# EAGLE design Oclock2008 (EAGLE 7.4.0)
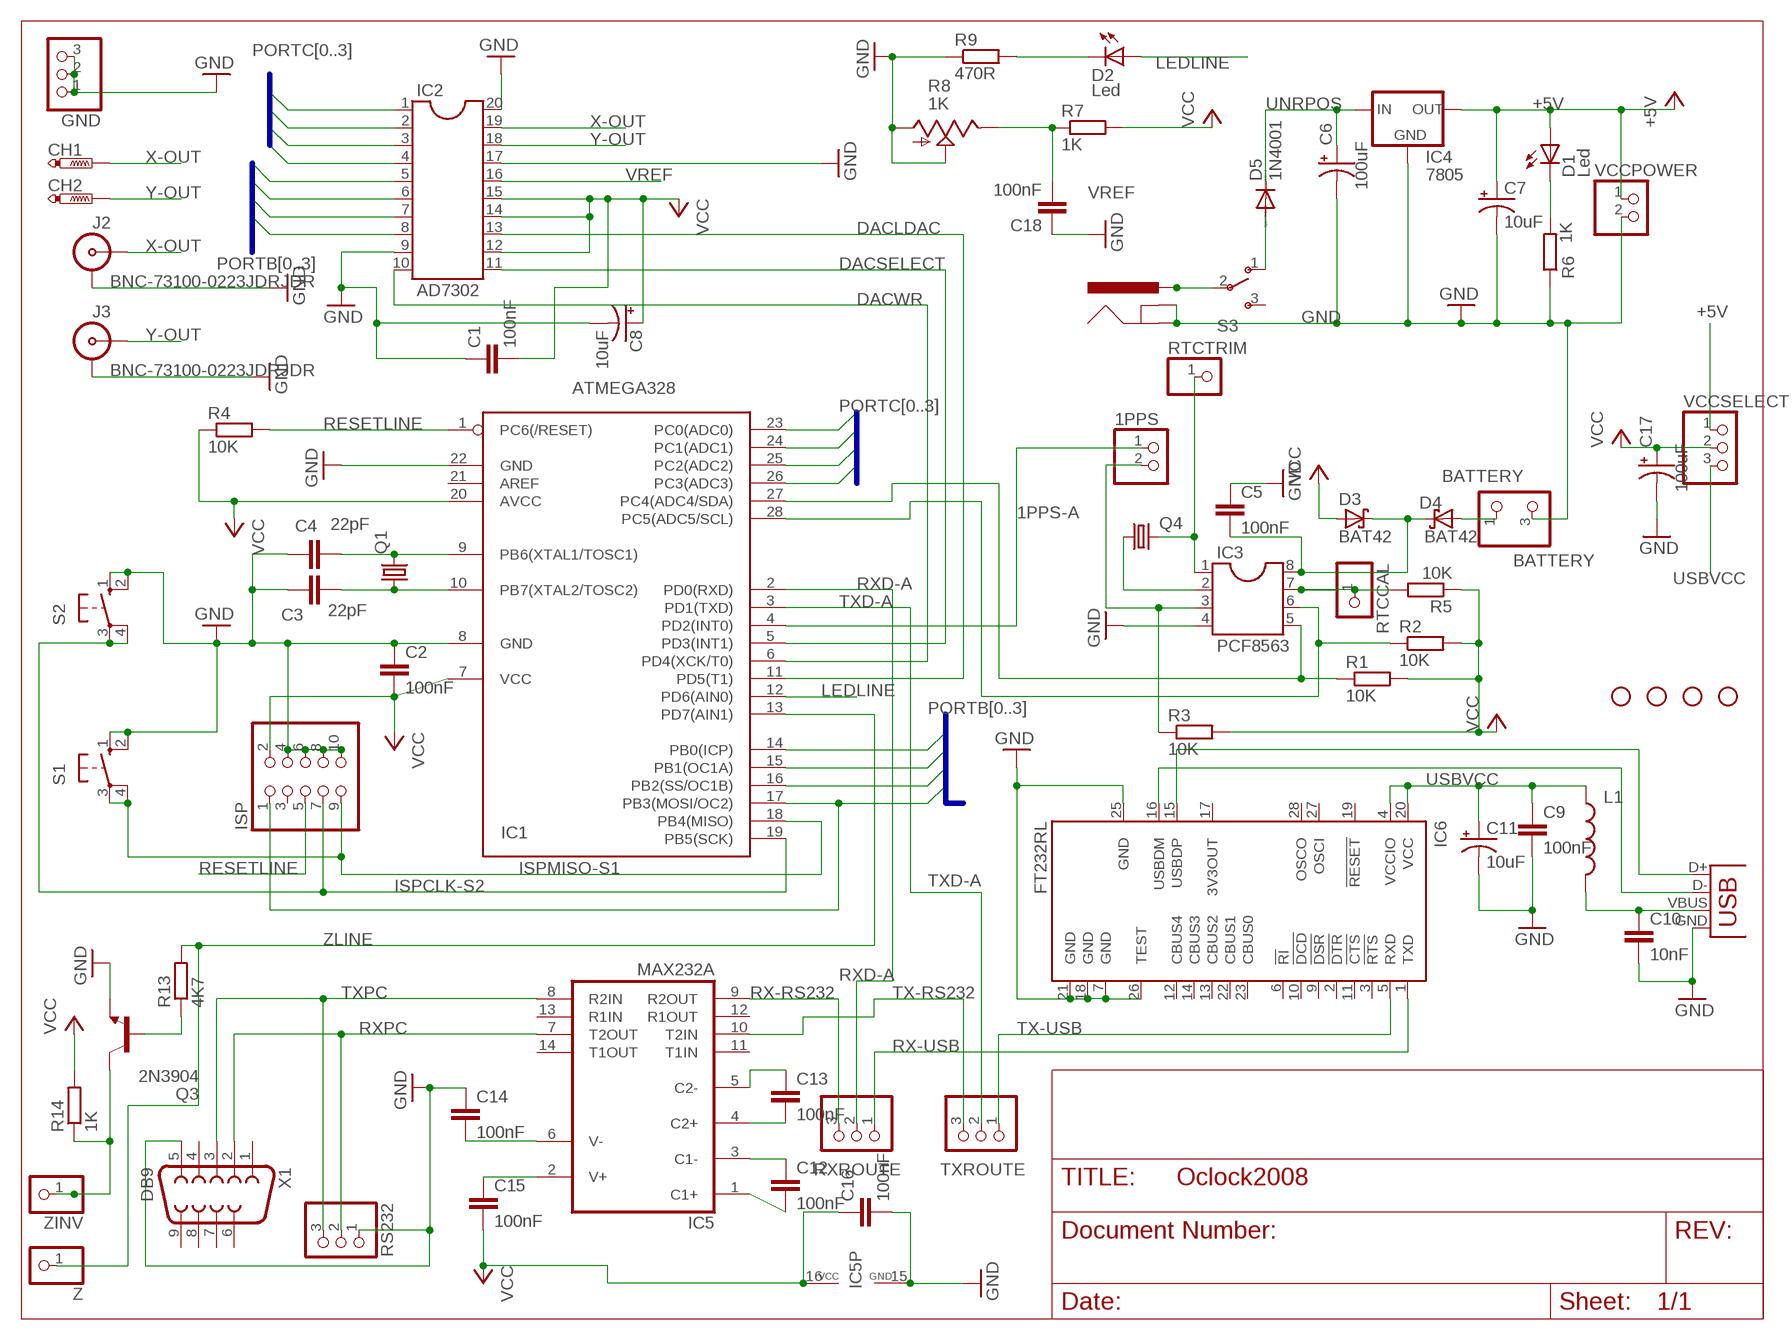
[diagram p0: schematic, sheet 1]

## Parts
1PPS  PINHD-1X2  [1X02]
BATTERY  BATTERY  PINHD-1X3BAT  [1X03BAT]
C1  100nF  C-EU025-025X050  [C025-025X050]
C2  100nF  C-EU025-025X050  [C025-025X050]
C3  22pF  C-EU025-025X050  [C025-025X050]
C4  22pF  C-EU025-025X050  [C025-025X050]
C5  100nF  C-EU025-025X050  [C025-025X050]
C6  100uF  CPOL-USE2.5-7  [E2,5-7]
C7  10uF  CPOL-USE2.5-5  [E2,5-5]
C8  10uF  CPOL-USE2.5-5  [E2,5-5]
C9  100nF  CAP0603  [0603]
C10  10nF  CAP0603  [0603]
C11  10uF  CAP_POL3528  [EIA3528]
C12  100nF  C-EU025-025X050  [C025-025X050]
C13  100nF  C-EU025-025X050  [C025-025X050]
C14  100nF  C-EU025-025X050  [C025-025X050]
C15  100nF  C-EU025-025X050  [C025-025X050]
C16  100nF  C-EU025-025X050  [C025-025X050]
C17  100uF  CPOL-USE2.5-7  [E2,5-7]
C18  100nF  C-EU025-025X050  [C025-025X050]
CH1  PTR1PAD1-20Y  [P1-20Y]
CH2  PTR1PAD1-20Y  [P1-20Y]
D1  Led  LED3MM  [LED3MM]
D2  Led  LED3MM  [LED3MM]
D3  BAT42  SCHOTTKY-DIODEDO35-7  [DO35-7]
D4  BAT42  SCHOTTKY-DIODEDO35-7  [DO35-7]
D5  1N4001  1N4004  [DO41-10]
GND  PINHD-1X3  [1X03]
IC1  ATMEGA328  MEGA8-P  [DIL28-3]
IC2  AD7302  DIL20  [DIL20]
IC3  PCF8563  DIL8  [DIL08]
IC4  7805  V_REG_78XXSINK  [TO220-IGO]
IC5  MAX232A  MAX232  [DIL16]
IC6  FT232RL  [SSOP28]
ISP  PINHD-2X5  [2X05]
J1  POWER_JACKPTH  [POWER_JACK_PTH]
J2  BNC-73100-0223JDRJDR  [73100-0223JDR]
J3  BNC-73100-0223JDRJDR  [73100-0223JDR]
L1  INDUCTOR0603  [0603]
Q1  CRYSTALHC18U-V  [HC18U-V]
Q3  2N3904  [TO92]
Q4  CRYSTALTC26H  [TC26H]
R1  10K  R-EU_0207/10  [0207/10]
R2  10K  R-EU_0207/10  [0207/10]
R3  10K  R-EU_0207/10  [0207/10]
R4  10K  R-EU_0207/10  [0207/10]
R5  10K  R-EU_0207/10  [0207/10]
R6  1K  R-EU_0207/10  [0207/10]
R7  1K  R-EU_0207/10  [0207/10]
R8  1K  TRIM_US-LI10  [LI10]
R9  470R  R-EU_0207/10  [0207/10]
R13  4K7  R-EU_0207/10  [0207/10]
R14  1K  R-EU_0207/10  [0207/10]
RS232  PINHD-1X3  [1X03]
RTCCAL  PINHD-1X1  [1X01]
RTCTRIM  PINHD-1X1  [1X01]
RXROUTE  PINHD-1X3  [1X03]
S1  10-XX  [B3F-10XX]
S2  10-XX  [B3F-10XX]
S3  SWITCH-SPSTPTH  [SWITCH-SPST]
TXROUTE  PINHD-1X3  [1X03]
U$2  STAND-OFF  [STAND-OFF]
U$3  STAND-OFF  [STAND-OFF]
U$4  STAND-OFF  [STAND-OFF]
U$5  STAND-OFF  [STAND-OFF]
VCCPOWER  PINHD-1X2  [1X02]
VCCSELECT  PINHD-1X3  [1X03]
X1  DB9  [DB9]
X2  USBPTH  [USB-B-PTH]
Z  PINHD-1X1  [1X01]
ZINV  PINHD-1X1  [1X01]

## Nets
1PPS-A: 1PPS.1 IC1.4(PD2(INT0))
1PPS-B: 1PPS.2 IC3.3 R3.1
+5V: C7.+ D1.A IC4.OUT VCCPOWER.1 VCCSELECT.1
BATPOWER: BATTERY.1 D4.A
DACLDAC: IC1.11(PD5(T1)) IC2.13
DACSELECT: IC1.5(PD3(INT1)) IC2.11
DACWR: IC1.6(PD4(XCK/T0)) IC2.10
GND: BATTERY.3 C1.1 C2.1 C3.2 C4.2 C5.1 C6.- C7.- C8.- C9.2 C10.2 C11.C(-) C14.1 C16.2 C17.- C18.1 GND.1 GND.2 GND.3 IC1.8(GND) IC1.22(GND) IC2.9 IC2.17 IC2.20 IC3.4 IC4.GND IC5.15(GND) IC6.7(GND) IC6.18(GND) IC6.21(GND) IC6.25(GND) IC6.26(TEST) ISP.4 ISP.6 ISP.8 ISP.10 J1.GND J1.GNDBREAK J2.GND J3.GND Q3.3(E) R6.1 R8.A R8.S R9.1 RS232.1 S1.1(S) S1.2(S1) S2.1(S) S2.2(S1) VCCPOWER.2 X1.5 X2.GND
ISPCLK-S2: IC1.19(PB5(SCK)) ISP.7 S2.3(P) S2.4(P1)
ISPMISO-S1: IC1.18(PB4(MISO)) ISP.9 S1.3(P) S1.4(P1)
LEDLINE: D2.A IC1.12(PD6(AIN0))
N$1: IC3.7 R5.2 RTCCAL.1
N$2: J1.PWR S3.2(P)
N$3: D2.K(C) R9.2
N$6: D1.K(C) R6.2
N$7: D5.A S3.1(O)
N$8: C13.2 IC5.4(C2+)
N$11: C4.1 IC1.9(PB6(XTAL1/TOSC1)) Q1.2
N$12: C3.1 IC1.10(PB7(XTAL2/TOSC2)) Q1.1
N$13: IC3.1 Q4.2 RTCTRIM.1
N$14: IC3.2 Q4.1
N$15: C13.1 IC5.5(C2-)
N$20: C12.1 IC5.3(C1-)
N$21: C12.2 IC5.1(C1+)
N$22: C14.2 IC5.6(V-)
N$23: C15.1 IC5.2(V+)
N$26: Q3.2(B) R13.1
PORTB0: IC1.14(PB0(ICP)) IC2.8
PORTB1: IC1.15(PB1(OC1A)) IC2.7
PORTB2: IC1.16(PB2(SS/OC1B)) IC2.6
PORTB3: IC1.17(PB3(MOSI/OC2)) IC2.5 ISP.1
PORTC0: IC1.23(PC0(ADC0)) IC2.4
PORTC1: IC1.24(PC1(ADC1)) IC2.3
PORTC2: IC1.25(PC2(ADC2)) IC2.2
PORTC3: IC1.26(PC3(ADC3)) IC2.1
RESETLINE: IC1.1(PC6(/RESET)) ISP.5 R4.2
RTCPOWER: C5.2 D3.C D4.C IC3.8
RX-RS232: IC5.9(R2OUT) RXROUTE.3
RX-USB: IC6.1(TXD) RXROUTE.1
RXD-A: IC1.2(PD0(RXD)) RXROUTE.2
RXPC: IC5.7(T2OUT) RS232.2 X1.2
SCLLINE: IC1.28(PC5(ADC5/SCL)) IC3.6 R2.1
SDALINE: IC1.27(PC4(ADC4/SDA)) IC3.5 R1.1
TX-RS232: IC5.10(T2IN) TXROUTE.3
TX-USB: IC6.5(RXD) TXROUTE.1
TXD-A: IC1.3(PD1(TXD)) TXROUTE.2
TXPC: IC5.8(R2IN) RS232.3 X1.3
UNRPOS: C6.+ D5.C IC4.IN
USB5V: C10.1 L1.2 X2.VBUS
USBDM: IC6.16(USBDM) X2.D-
USBDP: IC6.15(USBDP) X2.D+
USBVCC: C9.1 C11.A(+) IC6.4(VCCIO) IC6.20(VCC) L1.1 VCCSELECT.3
VCC: C1.2 C2.2 C8.+ C15.2 C16.1 C17.+ D3.A IC1.7(VCC) IC1.20(AVCC) IC2.12 IC2.14 IC2.15 IC5.16(VCC) ISP.2 R1.2 R2.2 R3.2 R4.1 R5.1 R7.2 R14.2 VCCSELECT.2
VREF: C18.2 IC2.16 R7.1 R8.E
X-OUT: CH1.TP IC2.19 J2.P
Y-OUT: CH2.TP IC2.18 J3.P
ZINVLINE: Q3.1(C) R14.1 ZINV.1
ZLINE: IC1.13(PD7(AIN1)) R13.2 Z.1
Unconnected: IC1.21(AREF) IC5.11(T1IN) IC5.12(R1OUT) IC5.13(R1IN) IC5.14(T1OUT) IC6.2(!DTR) IC6.3(!RTS) IC6.6(!RI) IC6.9(!DSR) IC6.10(!DCD) IC6.11(!CTS) IC6.12(CBUS4) IC6.13(CBUS2) IC6.14(CBUS3) IC6.17(3V3OUT) IC6.19(!RESET) IC6.22(CBUS1) IC6.23(CBUS0) IC6.27(OSCI) IC6.28(OSCO) ISP.3 S3.3(S) X1.1 X1.4 X1.6 X1.7 X1.8 X1.9

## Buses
PORTC[0..3]
PORTB[0..3]

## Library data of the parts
1PPS VCCPOWER = pinhead:PINHD-1X2: PIN HEADER
BATTERY = pinhead:PINHD-1X3BAT
C1-C5 C12-C16 C18 = rcl:C-EU: CAPACITOR, European symbol
C6-C8 C17 = rcl:CPOL-US: POLARIZED CAPACITOR, American symbol
C9 C10 = SparkFun:CAP: Capacitor
C11 = SparkFun:CAP_POL: Capacitor Polarized
CH1 CH2 = testpad:PTR1: TEST PIN
D1 D2 = led:LED: LED
D3 D4 = diode:SCHOTTKY-DIODE: Schottky Diode
D5 = diode:1N4004: DIODE
GND RS232 RXROUTE TXROUTE VCCSELECT = pinhead:PINHD-1X3: PIN HEADER
IC1 = atmel:MEGA8-P: MICROCONTROLLER 8 Kbytes FLASH, 1 kbytes SRAM, 512 bytes EEPROM, USART, 4-channel 10 bit ADC, 2-channel 8 bit ADC Pin compatible with Atmega48, ATMega88, ATMega168 Source: avr.lbr; OC_FARNELL: unknown; OC_NEWARK: unknown
IC2 = ic-package:DIL20: Dual In Line / Socket
IC3 = ic-package:DIL8: Dual In Line / Socket
IC4 = SparkFun:V_REG_78XX: Voltage Regulator Standard 7805 5V regulator. IGO (Input Ground Output). Spark Fun Electronics SKU : COM-00107
IC5 = maxim:MAX232: RS232 TRANSCEIVER; MF: MAXIM; MPN: MAX232ACPE+; OC_FARNELL: 9723773; OC_NEWARK: 68K4544
IC6 = ftdichip:FT232R: Source: http://www.ftdichip.com/Documents/DataSheets/DS_FT232R_v104.pdf; MPN: FT232RL; OC_FARNELL: 1146032; OC_NEWARK: 91K9918
ISP = pinhead:PINHD-2X5: PIN HEADER
J1 = SparkFun:POWER_JACK: Power Jack This is the standard 5.5mm barrel jack for power. The PTH is the most common, proven, reliable, footprint. All others are experimental. The Slot footprint only works if the mill layer is transmitted to the PCB fab house so be warned. Spark Fun Electronics SKU : PRT-00119. Mating wall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
J2 J3 = Jdr-Eagle:BNC-73100-0223JDR
L1 = SparkFun:INDUCTOR: Inductors
Q1 Q4 = crystal:CRYSTAL: CRYSTAL; OC_FARNELL: unknown; OC_NEWARK: unknown
Q3 = transistor-npn:2N3904: NPN Transistor
R1-R7 R9 R13 R14 = rcl:R-EU_: RESISTOR, European symbol
R8 = pot:TRIM_US-: POTENTIOMETER
RTCCAL RTCTRIM Z ZINV = pinhead:PINHD-1X1: PIN HEADER
S1 S2 = switch-omron:10-XX: OMRON SWITCH; MPN: B3F-1000; OC_FARNELL: 176432; OC_NEWARK: 36M3542
S3 = SparkFun:SWITCH-SPST: SPST Switch Simple slide switch. Spark Fun Electronics SKU : COM-00102
U$2-U$5 = SparkFun:STAND-OFF: Stand Off
X1 = SparkFun:DB9: DB9 Connector Standard DB9 (D-Sub 9) serial connector. Can be used for CAN bus as well as RS485 and RS232. Footprint production proven. Spark Fun Electronics SKU : PRT-00429
X2 = SparkFun:USB: USB Connectors USB-B-PTH is fully proven SKU : PRT-00139 USB-miniB is fully proven SKU : PRT-00587 USB-A-PCB is untested. USB-A-H is throughly reviewed, but untested. Spark Fun Electronics SKU : PRT-00437 USB-B-SMT is throughly reviewed, but untested. Needs silkscreen touching up. USB-A-S has not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

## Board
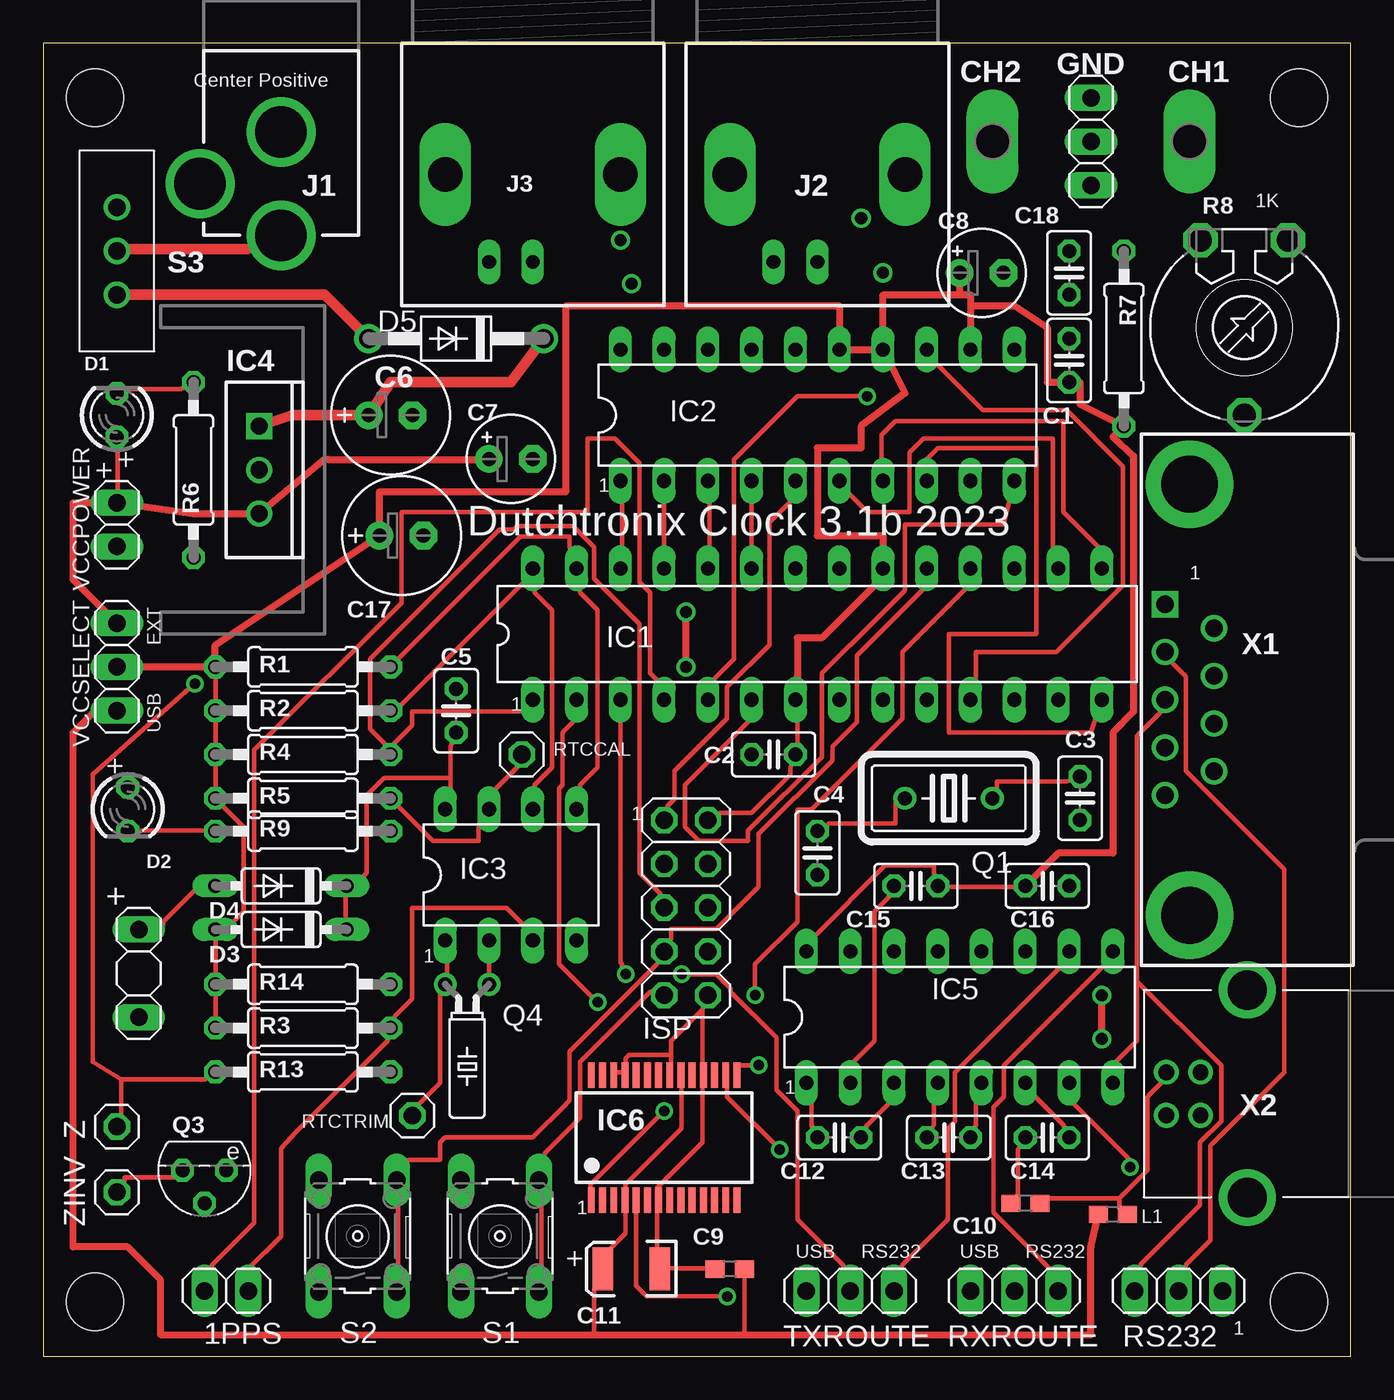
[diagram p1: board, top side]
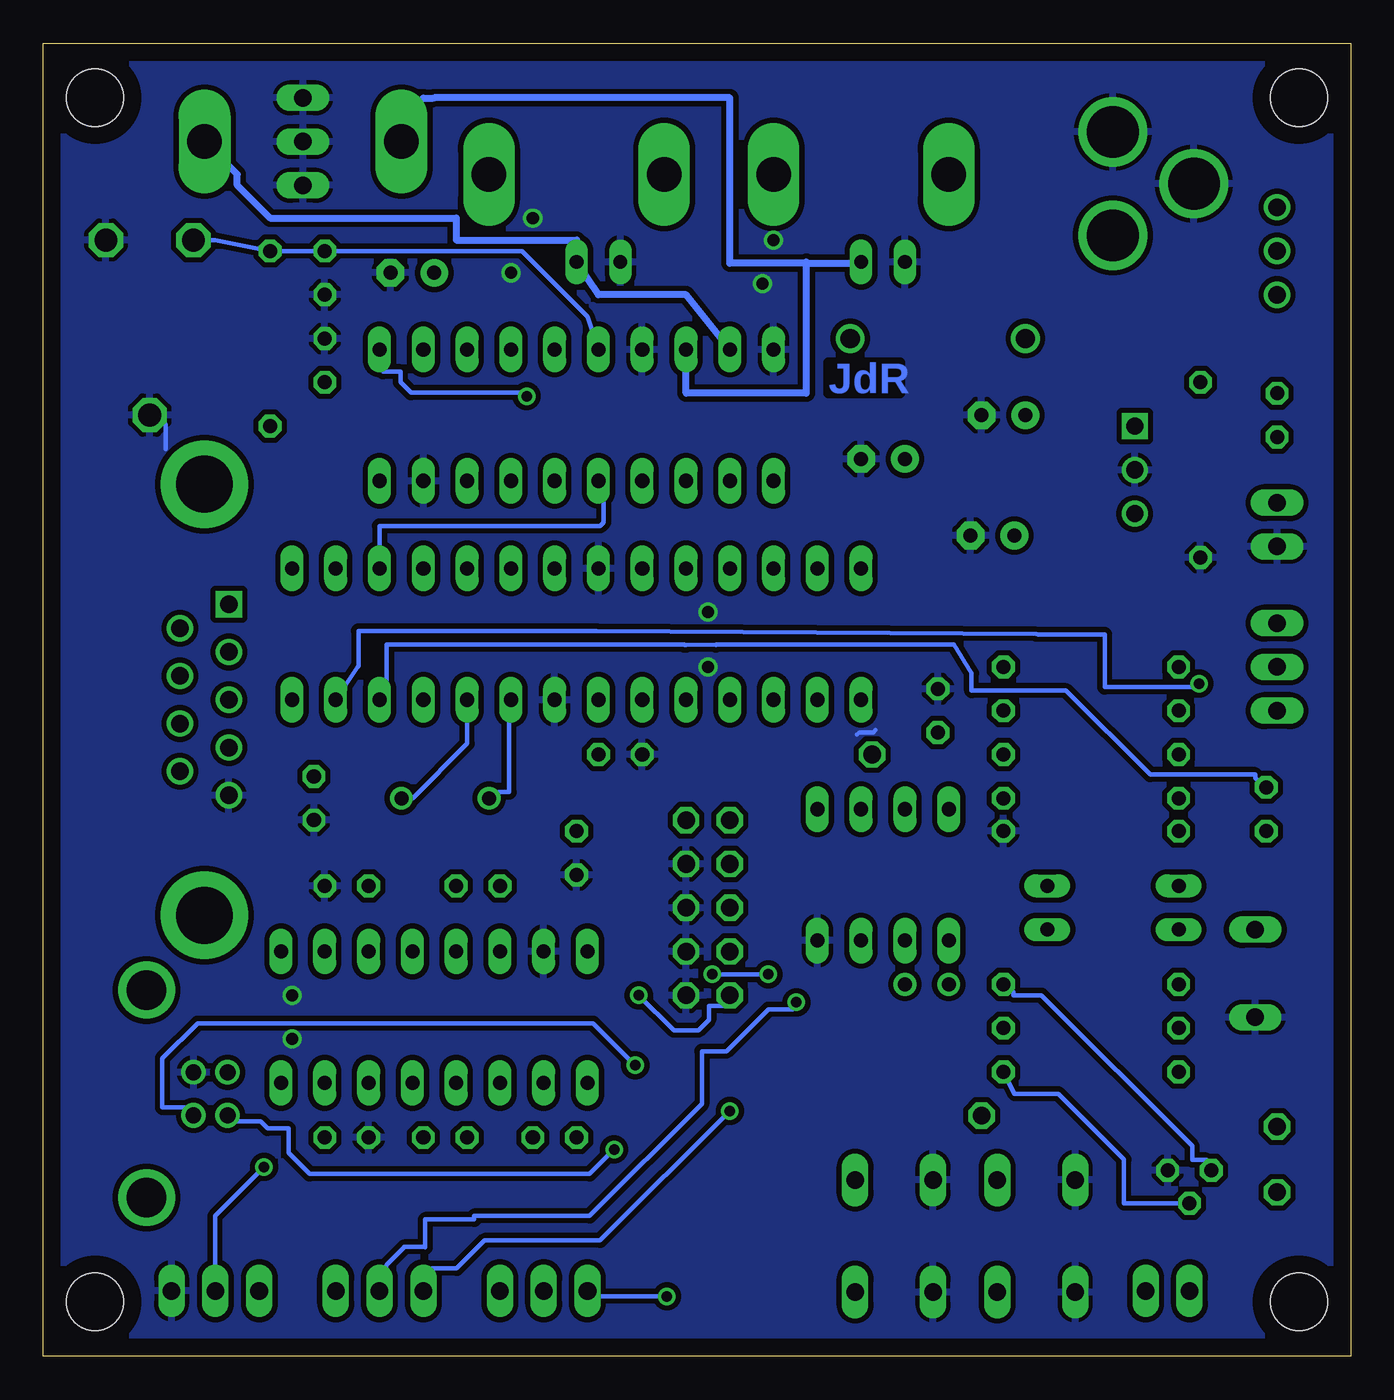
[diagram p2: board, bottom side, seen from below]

Size 75.87 x 76.19 mm. Coordinates in mm from the lower left corner, seen from the top.
Outline: 0,0 75.87,0 75.87,76.19 0,76.19 0,0
Copper layers (1*16): Top 0.035mm / dielectric 1.5mm / Bottom 0.035mm
Design rules "default *": minimum track width 10mil, minimum drill 24mil, track to track 8mil, track to pad 8mil, pad to pad 8mil, via to via 8mil, smd to smd 8mil, copper to edge 40mil, drill to drill 8mil, minimum pad ring 10mil, minimum via ring 8mil, stop-mask expansion 4mil, vias tented up to drill 0mil, thermal gap 10mil

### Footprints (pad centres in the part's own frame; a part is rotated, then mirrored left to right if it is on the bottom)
1X02 = drill 1.016 long: 1 -1.27,0; 2 1.27,0
1X03BAT = drill 1.016 long: 1 -2.54,0; 3 2.54,0
C025-025X050 = drill 0.813 octagon: 1 -1.27,0; 2 1.27,0
E2,5-7 = drill 0.813 pad 1.6: + -1.27,0 | drill 0.813 pad 1.6 octagon: - 1.27,0
E2,5-5 = drill 0.813 pad 1.6: + -1.27,0 | drill 0.813 pad 1.6 octagon: - 1.27,0
0603 = smd 1.1 x 1: 1 -0.85,0; 2 0.85,0
EIA3528 = smd 1.2 x 2.5: A 1.65,0; C -1.65,0
P1-20Y = drill 2.007 pad 2.54 long: TP 0,0
LED3MM = drill 0.813 octagon: A -1.27,0; K 1.27,0
DO35-7 = drill 0.813 long: A 3.81,0; C -3.81,0
DO41-10 = drill 1.118: A 5.08,0; C -5.08,0
1X03 = drill 1.016 long: 1 -2.54,0; 2 0,0; 3 2.54,0
DIL28-3 = drill 0.813 long: 1 -16.51,-3.81; 2 -13.97,-3.81; 3 -11.43,-3.81; 4 -8.89,-3.81; 5 -6.35,-3.81; 6 -3.81,-3.81; 7 -1.27,-3.81; 8 1.27,-3.81; 9 3.81,-3.81; 10 6.35,-3.81; 11 8.89,-3.81; 12 11.43,-3.81; 13 13.97,-3.81; 14 16.51,-3.81; 15 16.51,3.81; 16 13.97,3.81; 17 11.43,3.81; 18 8.89,3.81; 19 6.35,3.81; 20 3.81,3.81; 21 1.27,3.81; 22 -1.27,3.81; 23 -3.81,3.81; 24 -6.35,3.81; 25 -8.89,3.81; 26 -11.43,3.81; 27 -13.97,3.81; 28 -16.51,3.81
DIL20 = drill 0.813 long: 1 -11.43,-3.81; 2 -8.89,-3.81; 3 -6.35,-3.81; 4 -3.81,-3.81; 5 -1.27,-3.81; 6 1.27,-3.81; 7 3.81,-3.81; 8 6.35,-3.81; 9 8.89,-3.81; 10 11.43,-3.81; 11 11.43,3.81; 12 8.89,3.81; 13 6.35,3.81; 14 3.81,3.81; 15 1.27,3.81; 16 -1.27,3.81; 17 -3.81,3.81; 18 -6.35,3.81; 19 -8.89,3.81; 20 -11.43,3.81
DIL08 = drill 0.813 long: 1 -3.81,-3.81; 2 -1.27,-3.81; 3 1.27,-3.81; 4 3.81,-3.81; 5 3.81,3.81; 6 1.27,3.81; 7 -1.27,3.81; 8 -3.81,3.81
TO220-IGO = drill 1: GND 0,0; OUT 2.54,0 | drill 1 square: IN -2.54,0
DIL16 = drill 0.813 long: 1 -8.89,-3.81; 2 -6.35,-3.81; 3 -3.81,-3.81; 4 -1.27,-3.81; 5 1.27,-3.81; 6 3.81,-3.81; 7 6.35,-3.81; 8 8.89,-3.81; 9 8.89,3.81; 10 6.35,3.81; 11 3.81,3.81; 12 1.27,3.81; 13 -1.27,3.81; 14 -3.81,3.81; 15 -6.35,3.81; 16 -8.89,3.81
SSOP28 = smd 0.4 x 1.5: 1 -4.225,-3.625; 2 -3.575,-3.625; 3 -2.925,-3.625; 4 -2.275,-3.625; 5 -1.625,-3.625; 6 -0.975,-3.625; 7 -0.325,-3.625; 8 0.325,-3.625; 9 0.975,-3.625; 10 1.625,-3.625; 11 2.275,-3.625; 12 2.925,-3.625; 13 3.575,-3.625; 14 4.225,-3.625; 15 4.225,3.625; 16 3.575,3.625; 17 2.925,3.625; 18 2.275,3.625; 19 1.625,3.625; 20 0.975,3.625; 21 0.325,3.625; 22 -0.325,3.625; 23 -0.975,3.625; 24 -1.625,3.625; 25 -2.275,3.625; 26 -2.925,3.625; 27 -3.575,3.625; 28 -4.225,3.625
2X05 = drill 1.016 octagon: 1 -5.08,-1.27; 2 -5.08,1.27; 3 -2.54,-1.27; 4 -2.54,1.27; 5 0,-1.27; 6 0,1.27; 7 2.54,-1.27; 8 2.54,1.27; 9 5.08,-1.27; 10 5.08,1.27
POWER_JACK_PTH = drill 2.997: GND 0,7.7; GNDBREAK 4.7,10.7; PWR 0,13.7
73100-0223JDR = drill 0.8 long: GND 0,-1.27; P 0,1.27 | drill 2 long: GND1 -5.08,-3.81; P1 -5.08,6.35
HC18U-V = drill 0.813: 1 -2.54,0; 2 2.54,0
TO92 = drill 0.813 octagon: 1 1.27,0; 2 0,1.905; 3 -1.27,0
TC26H = drill 0.813: 1 -1.27,0; 2 1.27,0
0207/10 = drill 0.813 octagon: 1 -5.08,0; 2 5.08,0
LI10 = drill 1.321 octagon: A -2.54,-5.08; E 2.54,-5.08; S 0,5.08
1X01 = drill 1.016 octagon: 1 0,0
B3F-10XX = drill 1.016 long: 1 -3.251,2.261; 2 3.251,2.261; 3 -3.251,-2.261; 4 3.251,-2.261
SWITCH-SPST = drill 1.016: 1 0,2.54; 2 0,0; 3 0,-2.54
STAND-OFF = hole 3.302: 0,0
DB9 = drill 1.016 square: 1 -5.54,-1.42 | drill 1.016: 2 -2.77,-1.42; 3 0,-1.42; 4 2.77,-1.42; 5 5.54,-1.42; 6 -4.15,1.42; 7 -1.38,1.42; 8 1.38,1.42; 9 4.15,1.42 | drill 3.302 pad 5.08: G1 -12.5,0; G2 12.5,0
USB-B-PTH = drill 0.914: D+ 0,1.25; D- 1.981,1.25; GND 0,-1.25; VBUS 1.981,-1.25 | drill 2.286: P$1 -2.718,-6.02; P$2 -2.718,6.02

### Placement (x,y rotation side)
1PPS  10.63,3.8 0 top
BATTERY  5.55,22.22 270 top
C1  59.52,57.78 270 top
C2  42.38,34.92 0 top
C3  60.16,32.38 270 top
C4  44.92,29.2 270 top
C5  23.96,37.46 270 top
C6  20.15,54.61 0 top
C7  27.14,52.07 0 top
C8  54.45,62.86 0 top
C9  39.84,5.08 180 top
C10  56.98,8.89 180 top
C11  34.12,5.08 180 top
C12  46.19,12.7 180 top
C13  52.54,12.7 180 top
C14  58.25,12.7 0 top
C15  50.63,27.3 0 top
C16  58.25,27.3 0 top
C17  20.79,47.62 0 top
C18  59.52,62.86 90 top
CH1  66.51,70.48 180 top
CH2  55.08,70.48 0 top
D1  4.28,54.61 90 top
D2  4.92,31.74 270 top
D3  13.81,24.76 180 top
D4  13.81,27.3 180 top
D5  23.96,59.05 180 top
GND  60.8,70.48 270 top
IC1  44.92,41.91 0 top
IC2  44.92,54.61 0 top
IC3  27.14,27.93 0 top
IC4  12.54,51.43 270 top
IC5  53.17,19.68 0 top
IC6  36.03,12.7 0 top
ISP  37.3,26.03 270 top
J1  13.81,78.73 180 top
J2  43.65,63.5 270 top
J3  27.14,63.5 270 top
L1  62.06,8.25 0 top
Q1  52.54,32.38 180 top
Q3  9.36,10.79 180 top
Q4  24.6,21.58 180 top
R1  15.08,40 180 top
R2  15.08,37.46 180 top
R3  15.08,19.04 180 top
R4  15.08,34.92 0 top
R5  15.08,32.38 0 top
R6  8.73,51.43 90 top
R7  62.7,59.05 270 top
R8  69.69,59.69 180 top
R9  15.08,30.47 180 top
R13  15.08,16.5 180 top
R14  15.08,21.58 180 top
RS232  65.88,3.8 180 top
RTCCAL  27.77,34.92 0 top
RTCTRIM  21.42,13.97 0 top
RXROUTE  56.35,3.8 0 top
S1  26.5,6.98 90 top
S2  18.25,6.98 90 top
S3  4.28,64.13 180 top
TXROUTE  46.82,3.8 0 top
U$2  3.01,73.02 0 top
U$3  72.86,73.02 0 top
U$4  3.01,3.17 0 top
U$5  72.86,3.17 0 top
VCCPOWER  4.28,48.26 270 top
VCCSELECT  4.28,40 270 top
X1  66.51,38.1 270 top
X2  67.14,15.24 180 top
Z  4.28,13.33 270 top
ZINV  4.28,9.52 270 top

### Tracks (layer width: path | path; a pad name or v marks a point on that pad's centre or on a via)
1PPS-A
  Top 0.254: IC1.4 35.62,39.24 35.22,39.64 35.22,44.32 34.61,44.93 34.61,51.84 33.19,53.26 31.58,53.26 31.58,48.99 20.79,48.99 20.79,43.71 12.26,35.17 | 12.26,35.17 12.26,7.74 9.82,5.3 1PPS.1 | 12.26,35.17 12.26,35.2
1PPS-B
  Top 0.254: IC3.3 27.9,25.01 26.89,26.03 21.4,26.03 21.4,20.75 20.38,19.73 R3.1 19.98,18.31 14.69,13.03 13.81,12.06 13.81,6.98 11.9,5.08 1PPS.2
+5V
  Top 0.254: D1.A 4.33,52.65 4.33,50.21 VCCPOWER.1 | 25.26,52.04 C7.+ | 16.34,52.07 16.52,52.04
  Top 0.406: 16.52,52.04 25.26,52.04 | VCCSELECT.1 1.74,45.08 1.74,49.53 VCCPOWER.1 8.73,48.89 IC4.OUT 16.34,52.07
BATPOWER
  Top 0.254: D4.A 8.8,27.05 6.97,25.22 6.97,25.01 BATTERY.1
DACLDAC
  Top 0.254: IC2.13 51.88,57.53 54.52,54.88 59.4,54.88 62.65,51.63 62.65,44.72 58.79,40.86 54.12,40.86 54.12,39.44 IC1.11
DACSELECT  (via drill 0.61)
  Top 0.254: v47.82,55.7 43.75,55.7 40.09,52.04 40.09,40.46 38.88,39.24 IC1.5
  Bottom 0.254: v47.82,55.7 48.02,55.9 54.52,55.9 55.13,56.51 55.13,57.12 56.15,57.12 IC2.11
DACWR
  Top 0.254: IC2.10 55.71,48.26 50,48.26 50,44.45 46.82,41.27 46.8,41.27 45.17,39.64 45.17,34.77 40.91,30.5 40.91,29.89 38.06,29.89 37.25,30.7 37.25,33.14 40.91,36.8 IC1.6
GND  (via drill 0.7)
  Top 0.254: C10.2 56.55,9.37 56.55,12.01 C14.1 | C9.2 38.47,5.1 36.23,5.1 C11.C 35.62,6.32 35.62,8.35 IC6.7 35.62,9.77 38.27,12.42 38.27,15.67 IC6.18 38.27,16.89 38.27,20.14 | IC6.26 33.19,16.48 33.59,16.48 IC6.25 33.8,16.89 33.8,17.29 34,17.5 36.44,17.5 | 36.44,17.5 36.44,18.31 38.27,20.14 | 36.44,17.5 36.44,16.89 IC6.21 | 38.27,20.14 ISP.10
  Top 0.406: v61.43,18.41 v61.43,20.95 | v37.3,40 v37.3,43.18
  Bottom 0.254: 27.59,36.35 27.7,36.19 28.51,36.19 28.65,36.08 | R8.S 69.15,54.48 68.75,54.07 68.75,53.87 68.75,52.65
  other vias: 34.12,62.23 33.49,64.77 47.46,66.03 48.73,62.86
  pour Bottom (isolate 0.305): 0.47,76.19 76.03,76.19 76.03,-0.01 -0.17,-0.01
ISPCLK-S2
  Top 0.254: IC1.19 51.07,44.52 47.21,40.66 47.21,36.8 45.78,35.38 45.78,34.56 41.52,30.3 41.52,27.25 39.08,24.81 36.44,24.81 36.44,24.2 ISP.7 35.62,22.78 30.54,17.7 30.54,14.85 30.34,14.65 30.31,14.6 28.41,12.7 23.33,12.7 23.23,12.62 23.02,12.42 23.02,11.4 21.2,11.4 S2.4 20.59,8.76 20.59,5.3 S2.3
ISPMISO-S1  (via drill 0.61)
  Top 0.254: S1.3 28.92,5.3 28.92,8.76 S1.4 29.12,11.81 31.15,13.84 31.15,17.09 35.22,21.15 ISP.9 | v41.31,20.95 41.31,22.78 43.75,25.22 43.75,31.72 44.56,31.72 49.85,37 49.85,40.86 53.5,44.52 IC1.18
  Bottom 0.254: v41.31,20.95 39.28,18.92 37.86,18.92 37.25,19.53 37.25,20.34 36.44,20.34 ISP.9
LEDLINE
  Bottom 0.254: IC1.12 55.94,39.24 55.94,41.3 38.67,41.3 38.67,41.27 38.57,41.27 36.84,41.3 | 36.84,41.3 23.02,41.3 22.01,39.64 22.01,38.63 16.52,38.63 11.65,33.75 5.55,33.75 5.55,33.55 D2.A | 36.84,41.3 36.84,41.27
N$1
  Top 0.254: RTCCAL.1 27.5,34.16 26.28,32.94 IC3.7 25.26,30.7 25.26,29.89 22.62,29.89 20.59,31.92 R5.2
N$2
  Top 0.61: S3.2 4.94,64.23 11.85,64.23 J1.PWR
N$3
  Top 0.254: R9.2 9.41,30.5 5.75,30.5 D2.K
N$6
  Top 0.254: R6.2 7.99,56.1 5.14,56.1 D1.K
N$7
  Top 0.61: S3.1 16.34,61.59 D5.A
N$8
  Top 0.254: IC5.4 51.68,14.65 51.68,13.43 C13.2
N$11
  Top 0.254: C4.1 45.58,30.91 49.44,30.91 49.44,32.13 Q1.2
  Bottom 0.254: IC1.9 48.83,36.8 48.83,32.74 49.44,32.74 Q1.2
N$12
  Top 0.254: C3.1 59.4,33.35 55.33,33.35 55.33,32.94 Q1.1
  Bottom 0.254: IC1.10 51.27,35.55 54.45,32.38 Q1.1
N$13
  Top 0.254: IC3.1 23.43,22.98 23.43,22.17 Q4.2 23.02,20.95 23.02,15.87 21.81,14.65 RTCTRIM.1
N$14
  Top 0.254: Q4.1 IC3.2
N$15
  Top 0.254: IC5.5 54.12,14.65 54.12,13.43 C13.1
N$20
  Top 0.254: IC5.3 49.03,14.65 47.82,13.43 C12.1
N$21
  Top 0.254: IC5.1 44.56,14.65 44.56,13.43 C12.2
N$22
  Top 0.254: IC5.6 57.57,15.06 59.2,13.43 C14.2
N$23
  Top 0.254: IC5.2 47,17.09 48.22,18.31 48.22,25.83 49.03,26.64 C15.1
N$26
  Bottom 0.254: R13.1 19.52,15.24 16.98,15.24 13.17,11.43 13.17,8.89 Q3.2
PORTB0
  Top 0.254: IC2.8 51.27,52.07 51.91,52.7 57.62,52.7 57.62,41.91 52.54,41.91 52.54,36.19 60.8,36.19 IC1.14
PORTB1
  Top 0.254: IC2.7 48.63,52.04 48.63,53.46 49.44,54.28 59.2,54.28 59.2,48.99 61.23,46.96 IC1.15
PORTB2
  Top 0.254: IC2.6 46.8,50.01 47.82,48.99 50.25,48.99 50.25,52.45 51.07,53.26 58.59,53.26 58.59,46.96 IC1.16
PORTB3
  Top 0.254: IC2.5 43.34,49.6 42.13,48.38 42.13,41.27 39.69,38.83 39.69,37 36.64,33.96 36.64,32.33 36.23,31.92 ISP.1
  Bottom 0.254: IC1.17 56.35,48.18 43.55,48.18 43.34,48.38 43.34,49.6 IC2.5
PORTC0
  Top 0.254: IC1.23 IC2.4
PORTC1
  Top 0.254: IC2.3 38.67,49.6 38.67,46.96 IC1.24
PORTC2
  Top 0.254: IC1.25 IC2.2
PORTC3
  Top 0.254: IC1.26 33.59,46.96 33.59,49.6 IC2.1
RESETLINE
  Top 0.254: IC1.1 27.9,37.41 21.4,37.41 21.4,36.6 20.38,35.58 R4.2 19.77,35.58 18.96,36.39 18.96,40.46 26.48,47.98 27.29,47.98 27.5,48.18 30.75,48.18 31.97,46.96 31.97,45.13 34.61,42.49 34.61,28.06 35.83,26.84 ISP.5
RTCPOWER
  Top 0.254: D3.C 17.54,25.22 17.54,26.84 D4.C 18.55,27.86 18.76,28.06 18.76,32.53 19.77,33.55 23.63,33.55 | 23.63,33.55 23.63,35.38 C5.2 | 23.63,33.55 23.63,32.94 IC3.8
RX-RS232
  Top 0.254: IC5.9 61.43,22.58 55.74,16.89 55.74,15.06 55.13,14.45 55.13,8.35 58.38,5.1 RXROUTE.3
RX-USB  (via drill 0.61)
  Top 0.254: v36.03,14.24 31.76,9.98 31.76,9.77 IC6.1
  Bottom 0.254: v36.03,14.24 43.55,6.73 50.25,6.73 51.88,5.1 53.3,5.1 RXROUTE.1
RXD-A  (via drill 0.61)
  Top 0.254: v32.17,20.54 29.93,22.78 29.93,32.94 30.14,33.14 30.14,36.19 30.75,36.8 IC1.2
  Bottom 0.254: 53.71,6.34 54.93,6.34 54.93,6.32 55.94,5.3 RXROUTE.2 | v32.17,20.54 32.37,20.14 33.8,20.14 36.23,17.7 37.66,17.7 37.66,14.65 44.16,8.15 50.86,8.15 50.86,7.95 53.71,7.95 53.71,6.34 | 53.71,6.34 53.71,6.32
RXPC  (via drill 0.61)
  Top 0.254: RS232.2 66.31,5.3 67.73,6.73 67.73,12.21 72,16.48 72,28.27 66.31,33.96 66.31,39.44 65.49,40.25 X1.2 | v63.06,10.99 63.06,11.4 59.8,14.65 IC5.7
  Bottom 0.254: v63.06,10.99 65.9,8.15 65.9,5.3 RS232.2
SCLLINE
  Top 0.254: IC3.6 28.51,33.14 29.53,34.16 29.53,43.3 28.51,44.32 IC1.28 27.9,44.93 20.79,37.82 R2.1
SDALINE
  Top 0.254: R1.1 20.59,40.46 27.7,47.57 30.54,47.57 30.54,46.96 IC1.27 31.15,44.32 32.17,43.3 32.17,34.16 31.15,33.14 IC3.5
TX-RS232
  Top 0.254: IC5.10 58.99,22.58 52.9,16.48 52.9,13.64 52.49,13.23 52.49,7.95 49.85,5.3 TXROUTE.3
TX-USB  (via drill 0.61)
  Top 0.254: v39.69,3.48 35.01,3.48 34.4,4.08 34.4,8.35 IC6.5
  Bottom 0.254: v39.69,3.48 43.55,3.48 TXROUTE.1
TXD-A  (via drill 0.61)
  Top 0.254: IC1.3 33.49,22.86 33.59,22.78 33.59,22.37 v33.8,22.17 | v37.05,22.17 39.08,22.17 39.89,21.36 39.89,21.15 42.53,18.51 42.53,15.46 43.75,14.24 43.75,7.95 46.39,5.3 TXROUTE.2
  Bottom 0.254: v37.05,22.17 v33.8,22.17
TXPC
  Top 0.254: 63.46,21.76 63.46,35.99 64.88,37.41 X1.3 | 63.46,21.76 63.46,18.31 62.24,17.09 IC5.8 | 63.46,21.76 68.34,16.89 68.34,13.64 67.12,12.42 67.12,8.76 63.66,5.3 RS232.3
UNRPOS
  Top 0.61: D5.C 27.14,56.51 20.15,56.51 C6.+ 14.44,54.61 IC4.IN
USB5V
  Top 0.254: 62.45,9.16 58.38,9.16 C10.1 | 62.45,9.16 62.45,8.55 L1.2 | 62.45,9.16 64.07,10.79 64.07,15.06 64.88,15.87 X2.VBUS
USBDM  (via drill 0.61)
  Top 0.254: v42.74,12.01 39.69,15.06 39.69,15.67 IC6.16
  Bottom 0.254: v42.74,12.01 44.16,10.59 60.41,10.59 61.63,11.81 61.63,13.23 62.85,13.23 63.26,13.64 64.68,13.64 X2.D-
USBDP  (via drill 0.61)
  Top 0.254: v41.52,16.89 40.3,16.89 IC6.15
  Bottom 0.254: v41.52,16.89 43.95,19.32 66.92,19.32 68.95,17.29 68.95,14.45 67.53,14.45 X2.D+
USBVCC
  Top 0.254: C9.1 40.7,3.48 40.7,1.27 | 31.97,1.27 31.97,3.88 C11.A 32.98,6.32 33.8,7.13 33.8,8.35 IC6.4 33.8,9.77 33.8,9.98 37.05,13.23 37.05,15.67 IC6.20
  Top 0.406: VCCSELECT.3 3.01,37.46 1.74,36.19 1.74,6.34 4.92,6.34 6.82,4.44 6.82,1.27 31.97,1.27 40.7,1.27 60.8,1.27 60.8,6.34 L1.1
VCC
  Top 0.254: R1.2 10.02,39.44 10.02,38.02 R2.2 10.02,36.8 10.02,35.58 R4.1 10.02,34.36 10.02,32.94 R5.1 10.43,31.92 11.65,30.7 11.65,25.83 11.04,25.22 D3.A 10.02,24.2 10.02,22.17 R14.2 10.02,20.95 10.02,19.73 R3.2 | IC5.16 44.77,24.4 48.83,28.47 51.68,28.47 51.68,28.06 C15.2 52.69,27.25 56.35,27.25 C16.1 | IC1.7 43.75,36.8 43.75,35.58 C2.2 43.34,34.16 43.34,33.75 41.11,31.52 39.28,31.52 ISP.2 | 53.81,61.59 53.91,61.59 | 30.31,50.16 30.34,50.21
  Top 0.406: IC1.7 43.75,39.44 43.75,41.68 45.17,41.68 48.22,44.72 IC1.20 48.73,47.62 44.92,47.62 44.92,52.7 47.46,52.7 47.46,53.97 50,55.88 IC2.14 | IC2.15 IC2.14 | VCCSELECT.2 R1.2 10,41.27 C17.+ 19.52,50.16 30.31,50.16 | IC2.15 46.19,60.96 30.34,60.96 30.34,50.21 | IC2.14 48.73,61.59 53.17,61.59 | 53.17,61.59 53.81,61.59 53.81,60.96 | 53.81,60.96 IC2.12 | C16.1 58.89,29.2 62.06,29.2 62.06,36.19 63.26,37.41 63.26,52.24 62.06,53.34 R7.2 60.16,55.24 60.16,56.51 C1.2 58.25,56.51 58.25,59.69 56.35,60.96 53.81,60.96 | 53.17,61.59 C8.+ | IC2.15 IC2.14
VREF
  Bottom 0.254: IC2.16 44.28,60.32 48.09,64.13 C18.2 R7.1 65.88,64.77 R8.E
X-OUT
  Bottom 0.406: CH1.TP 64.61,68.57 64.61,67.94 62.7,66.03 51.91,66.03 51.91,64.77 44.92,64.77 J2.P 43.65,61.59 38.57,61.59 IC2.19
Y-OUT
  Bottom 0.254: 53.81,72.97 53.91,72.97 | 28.41,63.42 J3.P
  Bottom 0.406: CH2.TP 55.08,71.75 53.81,73.02 53.81,72.97 53.3,72.97 53.17,73.02 36.03,73.02 36.03,63.42 31.58,63.42 | 31.58,63.42 31.58,63.5 | 31.58,63.42 31.58,55.88 38.57,55.88 IC2.18 | 31.58,63.42 28.41,63.42
ZINVLINE
  Top 0.254: Q3.1 7.58,10.38 4.74,10.38 4.74,10.18 ZINV.1
  Bottom 0.254: R14.1 19.57,21.15 19.57,20.95 17.95,20.95 9.21,12.21 9.21,11.4 8.39,11.4 Q3.1
ZLINE  (via drill 0.61)
  Top 0.254: 4.53,16.07 9.41,16.07 R13.2 | 4.53,16.07 4.53,14.04 Z.1 | 4.53,16.07 2.88,17.09 2.88,33.75 v8.8,39.04
  Bottom 0.254: IC1.13 57.62,40 57.57,40.05 57.57,42.08 43.75,42.08 18.25,41.91 18.15,41.88 14.29,41.88 14.29,38.83 9.21,38.83 v8.8,39.04

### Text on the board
Bottom: JdR
tNames: Center Positive | 1K | + | + | 1 | Dutchtronix Clock 3.1b 2023 | 1 | EXT | 1 | USB | + | 1 | + | 1 | 1 | e | 1 | USB | RS232 | USB | RS232 | + | 1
